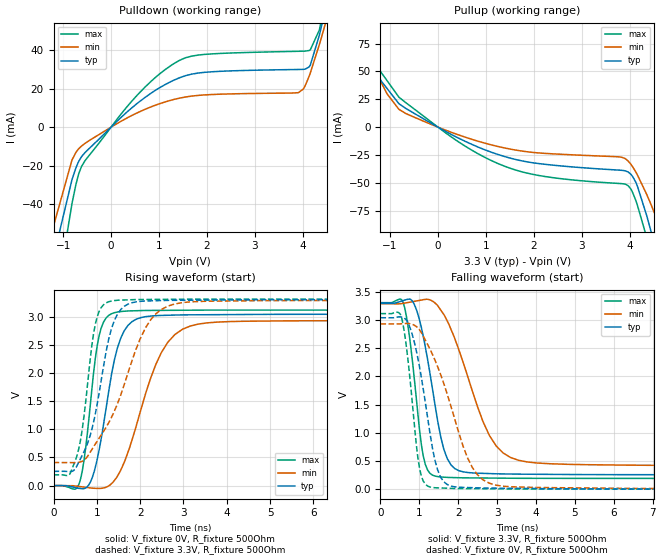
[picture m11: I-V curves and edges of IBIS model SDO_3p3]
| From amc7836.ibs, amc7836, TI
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|   Model
[Model]   SDO_3p3
Model_type   Output
Polarity   Non-Inverting
Vmeas = 1.65
Vref = 0
Cref = 1pF
Rref = 100000
|   typ   min   max
C_comp   2.780pF   2.357pF   3.166pF
[Voltage Range]   3.3   3.29   3.31
[Temperature Range]   27   125   -40
[Pullup Reference]   3.3   3.29   3.31
[Pulldown Reference]   0   0   0
[Power Clamp Reference]   3.3   3.29   3.31
[GND Clamp Reference]   0   0   0
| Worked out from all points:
|   slope of the pulldown table from 0 to 0.495 V, typ, clamps not added: 43.7 ohm
|   slope of the pullup table from 0 to 0.495 V, typ, clamps not added: 44.1 ohm
|   falling waveform, V_fixture 3.3V, R_fixture 500Ohm: 20-80 % time 467ps typ, 891ps min, 297ps max; typ from 3.3 V to 0.254 V
|   rising waveform, V_fixture 0V, R_fixture 500Ohm: 20-80 % time 426ps typ, 765ps min, 277ps max; typ from 0 V to 3.04 V
|   rising waveform, V_fixture 3.3V, R_fixture 500Ohm: 20-80 % time 471ps typ, 896ps min, 298ps max; typ from 0.254 V to 3.3 V
|   falling waveform, V_fixture 0V, R_fixture 500Ohm: 20-80 % time 444ps typ, 855ps min, 278ps max; typ from 3.04 V to 0 V
[Pulldown]
|   Voltage   I(typ)   I(min)   I(max)
-3.3V     -462mA     -322.2mA   -598.2mA
-1.241V   -78.92mA   -54.98mA   -106.4mA
-1.073V   -54.13mA   -40mA      -78.82mA
-815.1mV  -27.27mA   -17.09mA   -39.74mA
-617.1mV  -15.41mA   -9.855mA   -20.51mA
570.9mV   12.84mA    7.726mA    17.3mA
1.541V    26.65mA    15.61mA    35.94mA
3.907V    29.96mA    17.95mA    39.41mA
4.155V    32.26mA    28.18mA    40.19mA
4.372V    50.83mA    45.35mA    54.01mA
4.996V    121.8mA    99.73mA    143.2mA
6.6V      243mA      198.7mA    285.3mA
[Pullup]
|   Voltage   I(typ)   I(min)   I(max)
-3.3V     213mA      180.5mA    246.3mA
-1.815V   108.1mA    92.86mA    126.3mA
-1.062V   34.7mA     29.91mA    41.74mA
-676.5mV  16.97mA    12.37mA    22.16mA
570.9mV   -12.8mA    -9.044mA   -17.15mA
1.403V    -26.55mA   -18.81mA   -35.29mA
3.967V    -40.29mA   -30.47mA   -52.57mA
4.145V    -51.36mA   -41.7mA    -68.16mA
4.353V    -79.35mA   -60.34mA   -98.97mA
4.422V    -90.24mA   -67.29mA   -112.7mA
4.61V     -121.6mA   -87.36mA   -154.6mA
6.6V      -496.3mA   -348.9mA   -636.6mA
[Ramp]
R_load = 500
|   typ   min   max
dV/dt_r   1.82529/4.25495e-10   1.75955/7.64717e-10   1.86931/2.76689e-10
dV/dt_f   1.82789/4.66816e-10   1.7281/8.90544e-10   1.87171/2.97439e-10
[Falling Waveform]
V_fixture = 3.3V
V_fixture_min = 3.29V
V_fixture_max = 3.31V
R_fixture = 500Ohm
C_fixture = 0F
|   Time   V(typ)   V(min)   V(max)
0s        3.3V       3.29V      3.31V
590ps     3.347V     3.298V     3.305V
852.7ps   3.303V     3.331V     2.084V
1.099ns   2.719V     3.362V     596.3mV
1.404ns   1.497V     3.303V     232.5mV
1.631ns   707.7mV    3.099V     212.5mV
1.914ns   364.1mV    2.666V     205mV
2.8ns     276.8mV    954.6mV    197.2mV
3.548ns   266.8mV    513.2mV    193.1mV
20ns      253.5mV    409.8mV    190.5mV
[Rising Waveform]
V_fixture = 0V
V_fixture_min = 0V
V_fixture_max = 0V
R_fixture = 500Ohm
C_fixture = 0F
|   Time   V(typ)   V(min)   V(max)
0s        1.903uV    -6.422uV   231.6nV
590ps     -49.17mV   -15.36mV   30.54mV
704.7ps   -52.27mV   -26.48mV   454.5mV
852.7ps   65.45mV    -40.81mV   1.46V
1.099ns   831mV      -47.59mV   2.794V
1.486ns   2.467V     183.2mV    3.082V
1.815ns   2.912V     819.8mV    3.101V
2.488ns   3.02V      2.358V     3.109V
3.345ns   3.031V     2.866V     3.113V
20ns      3.042V     2.933V     3.116V
[Rising Waveform]
V_fixture = 3.3V
V_fixture_min = 3.29V
V_fixture_max = 3.31V
R_fixture = 500Ohm
C_fixture = 0F
|   Time   V(typ)   V(min)   V(max)
0s        253.6mV    409.7mV    190.5mV
494.2ps   290.5mV    407.7mV    426.2mV
637.3ps   500.4mV    424.6mV    871.3mV
773ps     723.9mV    507.3mV    1.707V
1.006ns   1.438V     786.4mV    2.991V
1.334ns   2.774V     1.206V     3.275V
1.631ns   3.181V     1.788V     3.294V
2.126ns   3.276V     2.803V     3.303V
2.977ns   3.289V     3.247V     3.307V
20ns      3.3V       3.29V      3.31V
[Falling Waveform]
|Gnd
V_fixture = 0V
V_fixture_min = 0V
V_fixture_max = 0V
R_fixture = 500Ohm
C_fixture = 0F
|   Time   V(typ)   V(min)   V(max)
0s        3.042V     2.933V     3.116V
536.3ps   3.055V     2.935V     3.066V
773ps     2.842V     2.934V     1.871V
1.006ns   2.166V     2.826V     369.8mV
1.271ns   1.005V     2.488V     39.09mV
1.472ns   338.8mV    2.173V     23.2mV
1.631ns   130.4mV    1.87V      19.2mV
2.362ns   26.42mV    385.8mV    9.274mV
2.977ns   17.75mV    70.19mV    5.687mV
20ns      -38.28uV   177uV      -161.2nV
